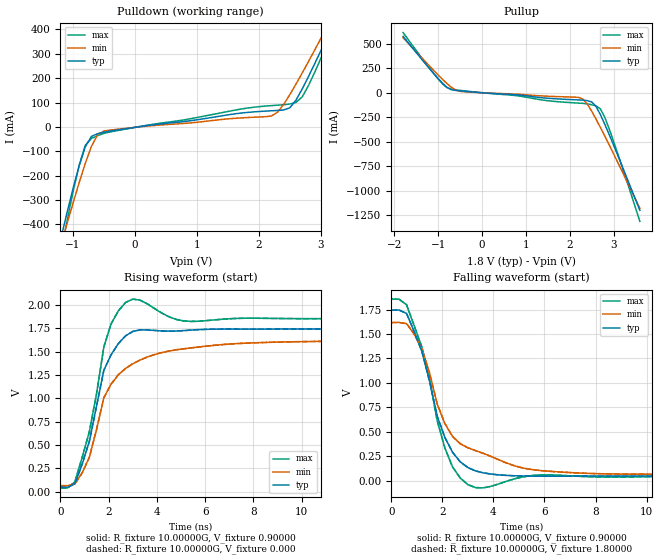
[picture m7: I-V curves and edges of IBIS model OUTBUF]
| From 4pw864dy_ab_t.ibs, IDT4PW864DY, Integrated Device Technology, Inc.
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|   Model OUTBUF
[Model]   OUTBUF
Model_type   Output
Polarity   Inverting
Vmeas =  0.90000V
C_comp   6.50000pF   5.40000pF   8.10000pF
[Temperature Range]   25.00000   0.11000k   0.000
[Voltage Range]   1.80000V   1.70000V   1.90000V
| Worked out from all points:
|   slope of the pulldown table from 0 to 0.27 V, typ, clamps not added: 28.1 ohm
|   slope of the pullup table from 0 to 0.27 V, typ, clamps not added: 33.1 ohm
|   rising waveform, R_fixture 10.00000G, V_fixture 0.90000: 20-80 % time 974ps typ, 1.42ns min, 824ps max; typ from 0.047 V to 1.74 V
|   rising waveform, R_fixture 10.00000G, V_fixture 0.000: 20-80 % time 974ps typ, 1.42ns min, 824ps max; typ from 0.047 V to 1.74 V
|   falling waveform, R_fixture 10.00000G, V_fixture 0.90000: 20-80 % time 1.14ns typ, 1.47ns min, 1ns max; typ from 1.74 V to 0.047 V
|   falling waveform, R_fixture 10.00000G, V_fixture 1.80000: 20-80 % time 1.14ns typ, 1.47ns min, 1ns max; typ from 1.74 V to 0.047 V
[Pulldown]
| voltage   I(typ)   I(min)   I(max)
-1.8V     -1.128A    -1.045A    -1.344A
-1.2V     -464.6mA   -492mA     -523.8mA
-1.1V     -358.4mA   -402.5mA   -393.5mA
-900mV    -160.8mA   -229.8mA   -158.6mA
-700mV    -39.01mA   -79.34mA   -47.05mA
-500mV    -21.55mA   -16.91mA   -26.61mA
2.2V      66.18mA    44.68mA    87.4mA
2.5V      78.51mA    132.7mA    94.2mA
2.7V      156.3mA    221.7mA    123.6mA
3.1V      366.9mA    410.7mA    340.2mA
3.2V      421.7mA    459mA      400.2mA
3.6V      643.8mA    653.9mA    644.4mA
[Pullup]
| voltage   I(typ)   I(min)   I(max)
-1.8V     578.6mA    564.8mA    617.5mA
-1.1V     197.3mA    229.2mA    198mA
-800mV    57.4mA     96.12mA    53.97mA
-500mV    20.69mA    15.96mA    25.67mA
2.2V      -71.71mA   -45.81mA   -104.5mA
2.3V      -74.17mA   -62.35mA   -107.1mA
2.5V      -91.56mA   -185.9mA   -120.9mA
2.6V      -137.5mA   -267.6mA   -133.6mA
2.7V      -222.2mA   -353.6mA   -163.6mA
2.8V      -321.1mA   -442.1mA   -250.1mA
3V        -533.4mA   -623.1mA   -494.8mA
3.6V      -1.202A    -1.18A     -1.314A
[Ramp]
| variable   typ   min   max
dV/dt_r   1.01819/0.97992n   0.93124/1.48763n   1.08925/0.80987n
dV/dt_f   1.01819/1.15580n   0.93181/1.53751n   1.08926/1.01402n
R_load = 10.00000G
[Rising Waveform]
R_fixture = 10.00000G
V_fixture = 0.90000
V_fixture_min = 0.85000
V_fixture_max = 0.95000
| time   V(typ)   V(min)   V(max)
0s        47.01mV    63.94mV    40.58mV
600ps     85.3mV     82.56mV    106.1mV
1.2ns     540.3mV    368.9mV    643.4mV
1.8ns     1.302V     1.007V     1.552V
2.1ns     1.468V     1.153V     1.8V
2.7ns     1.671V     1.321V     2.029V
3.3ns     1.735V     1.411V     2.054V
4.5ns     1.721V     1.508V     1.875V
5.4ns     1.732V     1.541V     1.825V
15ns      1.744V     1.616V     1.856V
[Rising Waveform]
R_fixture = 10.00000G
V_fixture = 0.000
V_fixture_min = 0.000
V_fixture_max = 0.000
| time   V(typ)   V(min)   V(max)
0s        47.01mV    63.94mV    40.58mV
600ps     85.3mV     82.56mV    106.1mV
1.2ns     540.3mV    368.9mV    643.4mV
1.8ns     1.302V     1.007V     1.552V
2.1ns     1.468V     1.153V     1.8V
2.7ns     1.671V     1.321V     2.029V
3.3ns     1.735V     1.411V     2.054V
4.5ns     1.721V     1.508V     1.875V
5.4ns     1.732V     1.541V     1.825V
15ns      1.744V     1.616V     1.856V
[Falling Waveform]
R_fixture = 10.00000G
V_fixture = 0.90000
V_fixture_min = 0.85000
V_fixture_max = 0.95000
| time   V(typ)   V(min)   V(max)
0s        1.744V     1.617V     1.856V
600ps     1.71V      1.606V     1.798V
1.2ns     1.321V     1.348V     1.365V
1.8ns     659.5mV    783.6mV    613.4mV
2.1ns     442.4mV    584.1mV    333.3mV
2.4ns     291.2mV    452.2mV    141.5mV
3ns       134.1mV    336.7mV    -40.38mV
3.6ns     80.11mV    279.6mV    -73.41mV
6ns       45.94mV    99.88mV    59.12mV
15ns      47.01mV    63.98mV    40.56mV
[Falling Waveform]
R_fixture = 10.00000G
V_fixture = 1.80000
V_fixture_min = 1.70000
V_fixture_max = 1.90000
| time   V(typ)   V(min)   V(max)
0s        1.744V     1.617V     1.856V
600ps     1.71V      1.606V     1.798V
1.2ns     1.321V     1.348V     1.365V
1.8ns     659.5mV    783.6mV    613.4mV
2.1ns     442.4mV    584.1mV    333.3mV
2.4ns     291.2mV    452.2mV    141.5mV
3ns       134.1mV    336.7mV    -40.38mV
3.6ns     80.11mV    279.6mV    -73.41mV
6ns       45.94mV    99.88mV    59.12mV
15ns      47.01mV    63.98mV    40.56mV
